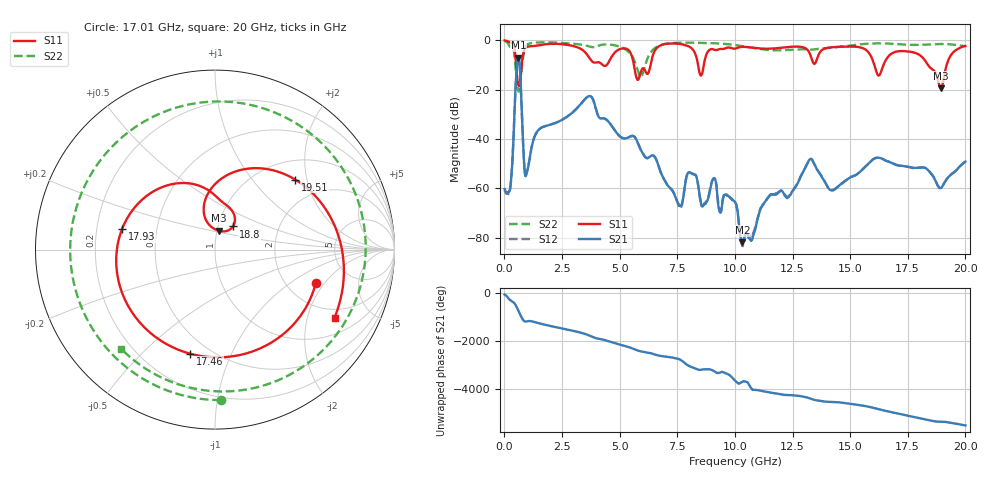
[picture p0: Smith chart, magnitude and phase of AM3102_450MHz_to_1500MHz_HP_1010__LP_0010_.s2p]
!Agilent Technologies,E8364B,MY43040894,A.07.50.67
!Agilent E8364B: A.07.50.67
!Date: Thursday, January 11, 2018 06:10:15
!Correction: S11(Full 2 Port(1,2))
!S21(Full 2 Port(1,2))
!S12(Full 2 Port(1,2))
!S22(Full 2 Port(1,2))
!S2P File: Measurements: S11, S21, S12, S22:
# Hz S  dB  R 50
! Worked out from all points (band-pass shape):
!   1601 points, 10 MHz to 20 GHz, reference 50 ohm
!   highest |S21| = -7.05 dB at 609.7 MHz (marker M1); lowest = -81.9 dB at 10.33 GHz (marker M2)
!   |S21| within 3 dB of the highest: 549.2 MHz to 664.9 MHz (115.6 MHz wide, 19 % of centre)
!   lowest |S11| = -19.4 dB at 18.94 GHz (marker M3), VSWR 1.24, Z = 51.2 + j10.8 ohm
!   |S11| at or under -10 dB: 5.62 GHz to 6.343 GHz (723.3 MHz wide, 12.1 % of centre); 16.05 GHz to 16.45 GHz (400.4 MHz wide, 2.46 % of centre); 18.38 GHz to 19.19 GHz (810.2 MHz wide, 4.31 % of centre)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
!   |S22| runs from -20.9 to -0.3 dB; largest |S21 - S12| = 0.00072
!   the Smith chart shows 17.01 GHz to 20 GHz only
!   S11 on the Smith chart (normalised r, x): 17.01 GHz: 2.86, -1.65; 17.46 GHz: 0.40, -0.71; 17.93 GHz: 0.31, +0.10; 18.8 GHz: 1.18, +0.31; 19.51 GHz: 1.42, +1.71; 20 GHz: 1.62, -2.97
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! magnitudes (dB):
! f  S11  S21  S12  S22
! 10 MHz  -0.1  -60.3  -60.8  -0.3
! 272.4 MHz  -0.9  -58.5  -58.3  -3.0
! 609.7 MHz  -18.3  -7.1  -7.1  -20.6
! 959.5 MHz  -2.8  -54.1  -54.1  -1.9
! 1.459 GHz  -2.1  -36.6  -36.6  -0.9
! 3.346 GHz  -3.6  -25.5  -25.5  -1.7
! 5.795 GHz  -16.0  -41.8  -41.7  -12.5
! 6.682 GHz  -2.6  -50.7  -50.8  -2.3
! 7.606 GHz  -1.5  -67.2  -68.1  -1.0
! 8.056 GHz  -2.8  -53.6  -53.6  -1.0
! 10.01 GHz  -3.4  -65.5  -65.5  -1.9
! 10.33 GHz  -2.7  -81.9  -83.3  -2.3
! 13.34 GHz  -7.8  -48.3  -48.4  -3.8
! 14.22 GHz  -2.8  -60.8  -60.8  -3.0
! 16.68 GHz  -6.4  -49.3  -49.2  -1.3
! 17.01 GHz  -4.6  -50.6  -50.5  -1.5
! 17.46 GHz  -4.5  -51.2  -51.2  -1.8
! 17.93 GHz  -5.5  -51.8  -51.6  -1.9
! 18.8 GHz  -15.8  -58.9  -58.9  -1.5
! 18.94 GHz  -19.4  -60.0  -59.6  -1.5
! 19.51 GHz  -4.5  -53.6  -53.4  -1.8
! 20 GHz  -2.3  -49.2  -49.2  -2.4
